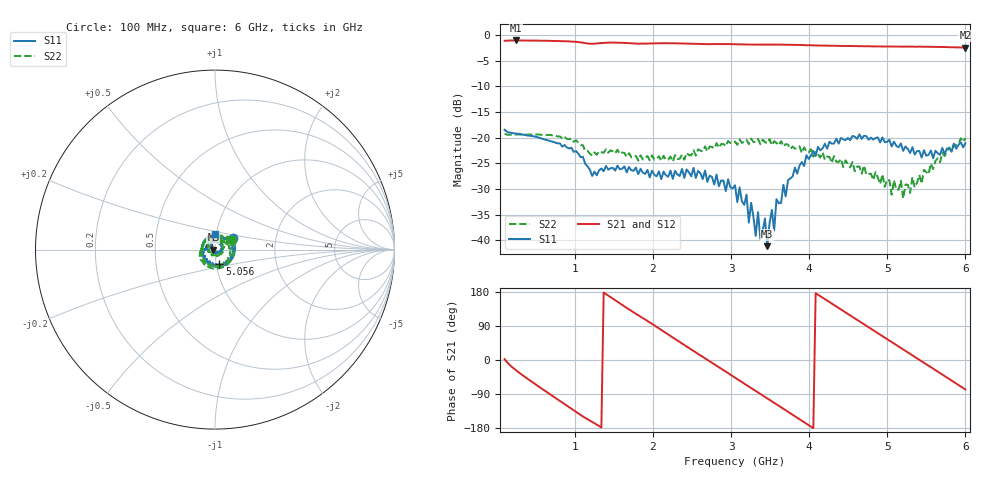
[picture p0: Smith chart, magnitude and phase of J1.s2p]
!Agilent Technologies,E8364B,MY43040379,A.07.50.67
!Agilent E8364B: A.07.50.67
!Date: Tuesday, March 24, 2026 11:34:31
!Correction: S11(Full 2 Port(1,2))
!S21(Full 2 Port(1,2))
!S12(Full 2 Port(1,2))
!S22(Full 2 Port(1,2))
!S2P File: Measurements: S11, S21, S12, S22:
# Hz S  dB  R 50
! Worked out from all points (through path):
!   201 points, 100 MHz to 6 GHz, reference 50 ohm
!   highest |S21| = -1.08 dB at 247.5 MHz (marker M1); lowest = -2.5 dB at 6 GHz (marker M2)
!   group delay of S21, straight-line fit = 370 ps
!   lowest |S11| = -41.1 dB at 3.463 GHz (marker M3), VSWR 1.02, Z = 49.1 + j0.0544 ohm
!   |S11| at or under -10 dB: start of sweep to end of sweep
!   |S22| runs from -31.8 to -19.2 dB; largest |S21 - S12| = 0.0027
!   S11 on the Smith chart (normalised r, x): 100 MHz: 1.21, +0.16; 5.056 GHz: 1.04, -0.16; 6 GHz: 0.98, +0.18
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1e8  -18.45 32.9  -1.15 2.2  -1.15 2.1  -19.24 29.6
2.475e8  -19.20 -15.8  -1.08 -27.3  -1.08 -27.5  -19.38 -17.8
6.605e8  -20.53 -90.1  -1.14 -87.5  -1.14 -87.6  -19.46 -91.9
1.103e9  -23.73 -175.3  -1.51 -149.0  -1.51 -149.1  -21.48 -170.9
1.5455e9  -25.44 138.7  -1.49 153.5  -1.49 153.5  -22.35 138.5
2.0765e9  -26.55 70.0  -1.62 83.4  -1.62 83.2  -23.59 73.3
2.578e9  -26.46 32.0  -1.77 16.2  -1.77 16.0  -22.26 32.4
3.05e9  -29.25 -31.4  -1.80 -46.5  -1.80 -46.7  -20.76 -32.1
3.1975e9  -31.09 -54.8  -1.85 -66.2  -1.85 -66.2  -20.39 -52.6
3.227e9  -36.53 -65.2  -1.87 -70.0  -1.87 -70.1  -21.26 -55.7
3.2565e9  -32.68 -54.7  -1.87 -73.8  -1.87 -73.9  -20.17 -58.2
3.3155e9  -39.11 -68.7  -1.89 -81.6  -1.89 -81.7  -20.80 -66.9
3.345e9  -34.49 -90.1  -1.88 -85.6  -1.89 -85.6  -20.22 -74.7
3.4335e9  -35.71 -153.9  -1.89 -97.3  -1.89 -97.3  -20.84 -92.8
3.463e9  -41.12 176.4  -1.89 -101.1  -1.89 -101.2  -21.08 -91.7
3.6695e9  -29.17 125.1  -1.90 -128.7  -1.89 -128.8  -21.69 -132.7
4.053e9  -22.59 65.6  -2.03 -179.9  -2.02 -179.9  -23.68 153.3
4.584e9  -19.81 -5.3  -2.17 110.0  -2.17 110.0  -26.53 37.6
5.0265e9  -20.42 -71.6  -2.25 51.8  -2.25 51.7  -28.28 -77.4
5.056e9  -21.71 -73.0  -2.26 47.8  -2.26 47.7  -31.11 -73.8
5.4985e9  -23.51 -166.8  -2.29 -11.0  -2.31 -11.1  -26.71 133.9
6e9  -21.07 90.2  -2.46 -77.7  -2.46 -77.7  -20.08 37.7
